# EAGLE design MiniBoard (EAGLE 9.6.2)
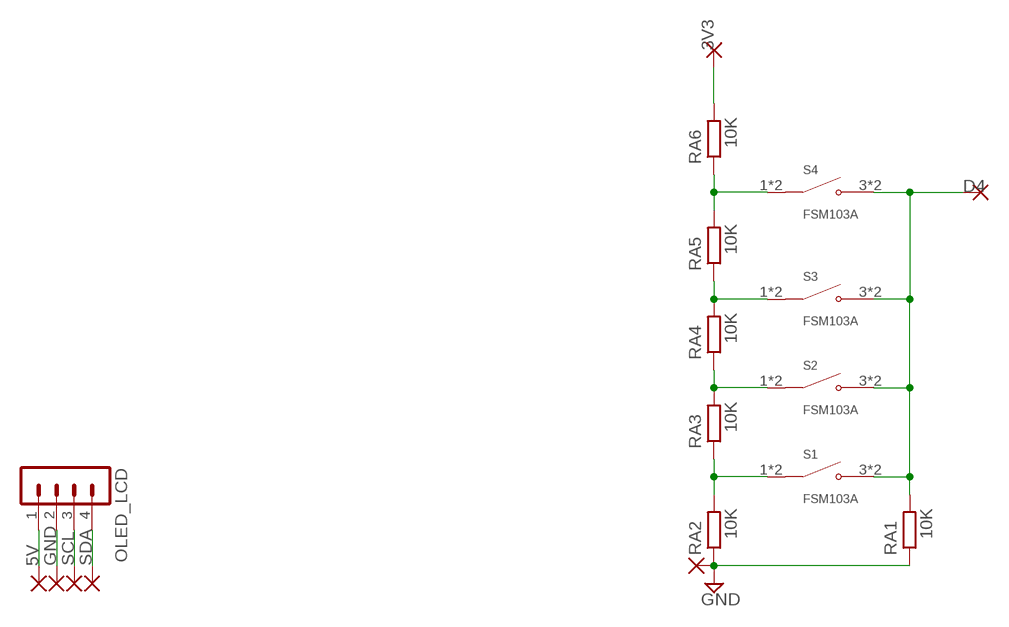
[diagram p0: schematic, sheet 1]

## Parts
OLED_LCD  MA04-1  [MA04-1]
PAD1  WIREPAD1,6/0,9  [1,6/0,9]
PAD25  WIREPAD1,6/0,9  [1,6/0,9]
PAD26  WIREPAD1,6/0,9  [1,6/0,9]
PAD52  WIREPAD1,6/0,9  [1,6/0,9]
PAD78  WIREPAD1,6/0,9  [1,6/0,9]
PAD103  WIREPAD1,6/0,9  [1,6/0,9]
PAD104  WIREPAD1,6/0,9  [1,6/0,9]
RA1  10K  R-EU_0309/12  [0309/12]
RA2  10K  R-EU_0309/12  [0309/12]
RA3  10K  R-EU_0309/12  [0309/12]
RA4  10K  R-EU_0309/12  [0309/12]
RA5  10K  R-EU_0309/12  [0309/12]
RA6  10K  R-EU_0309/12  [0309/12]
S1  FSM103A  [SW_1571627-1]
S2  FSM103A  [SW_1571627-1]
S3  FSM103A  [SW_1571627-1]
S4  FSM103A  [SW_1571627-1]

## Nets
3V3: PAD104.1(P) RA6.2
5V: OLED_LCD.1 PAD25.1(P)
D4: PAD103.1(P) RA1.2 S1.3(NO) S1.4(NO) S2.3(NO) S2.4(NO) S3.3(NO) S3.4(NO) S4.3(NO) S4.4(NO)
GND: OLED_LCD.2 PAD1.1(P) PAD26.1(P) RA1.1 RA2.1
N$5: RA4.2 RA5.1 S3.1(COM) S3.2(COM)
N$8: RA3.2 RA4.1 S2.1(COM) S2.2(COM)
N$9: RA2.2 RA3.1 S1.1(COM) S1.2(COM)
N$32: RA5.2 RA6.1 S4.1(COM) S4.2(COM)
SCL: OLED_LCD.3 PAD52.1(P)
SDA: OLED_LCD.4 PAD78.1(P)

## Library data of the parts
OLED_LCD = con-lstb:MA04-1: PIN HEADER; OC_FARNELL: unknown; OC_NEWARK: unknown
PAD1 PAD25 PAD26 PAD52 PAD78 PAD103 PAD104 = wirepad-ws:WIREPAD: Wire PAD connect wire on PCB
RA1-RA6 = rcl-ws:R-EU_: RESISTOR, European symbol; SPICEPREFIX: R
S1-S4 = FSM103A:FSM103A: Alcoswitch FSM100-104, Tactile Switches, Round Actuator Style, Operating Function NO, Brass Contact Base Material Check availability; AVAILABILITY: In Stock; CHECK_PRICES: https://www.snapeda.com/parts/FSM103A/TE+Connectivity+ALCOSWITCH+Switches/view-part/?ref=eda; COMMENT: 1571627-1; DESCRIPTION: Alcoswitch, Tactile switch,PCB,SPST,red actuator | TE Connectivity FSM103A; MF: TE Connectivity; MP: FSM103A; PACKAGE: None; PRICE: None; SNAPEDA_LINK: https://www.snapeda.com/parts/FSM103A/TE+Connectivity+ALCOSWITCH+Switches/view-part/?ref=snap

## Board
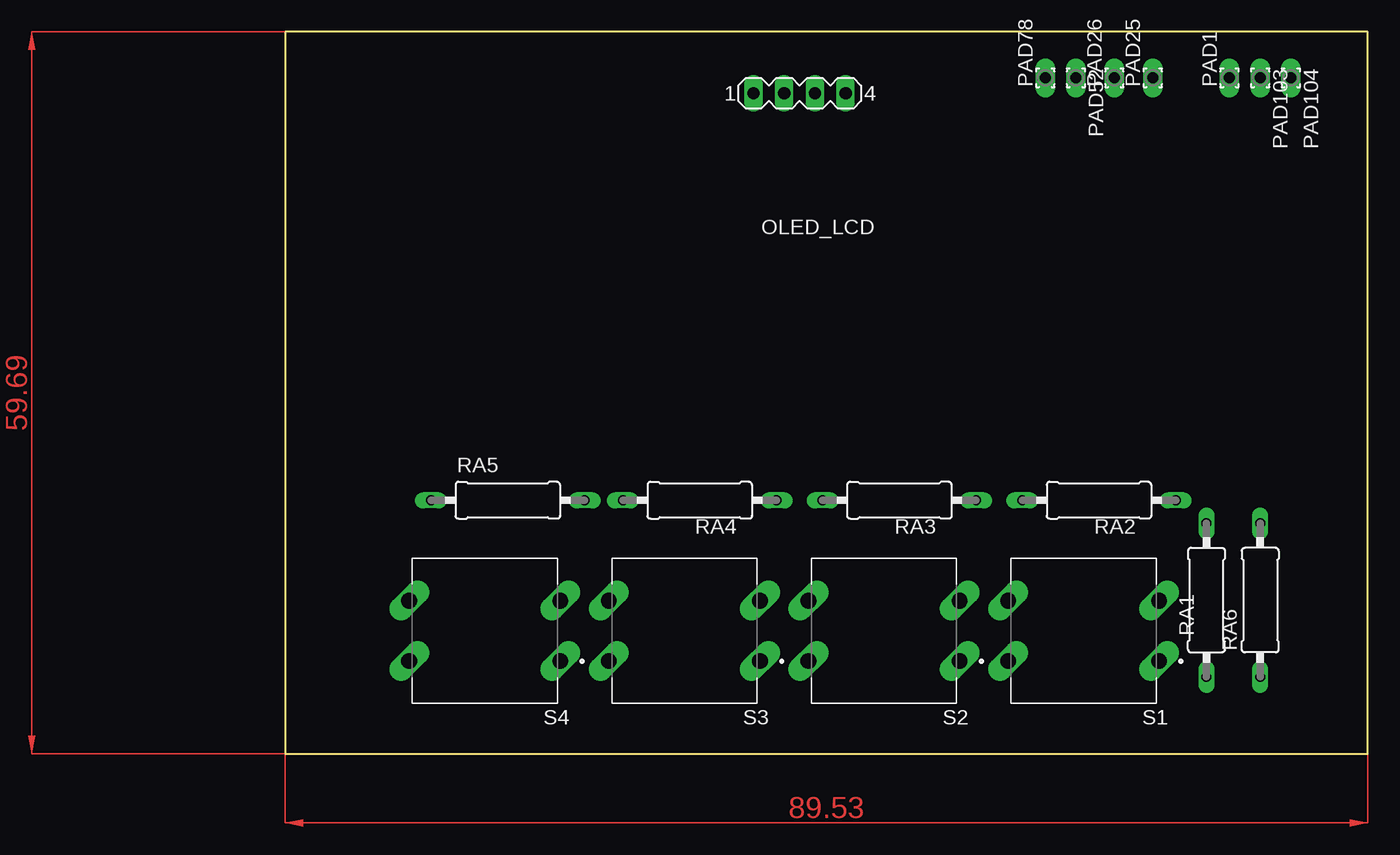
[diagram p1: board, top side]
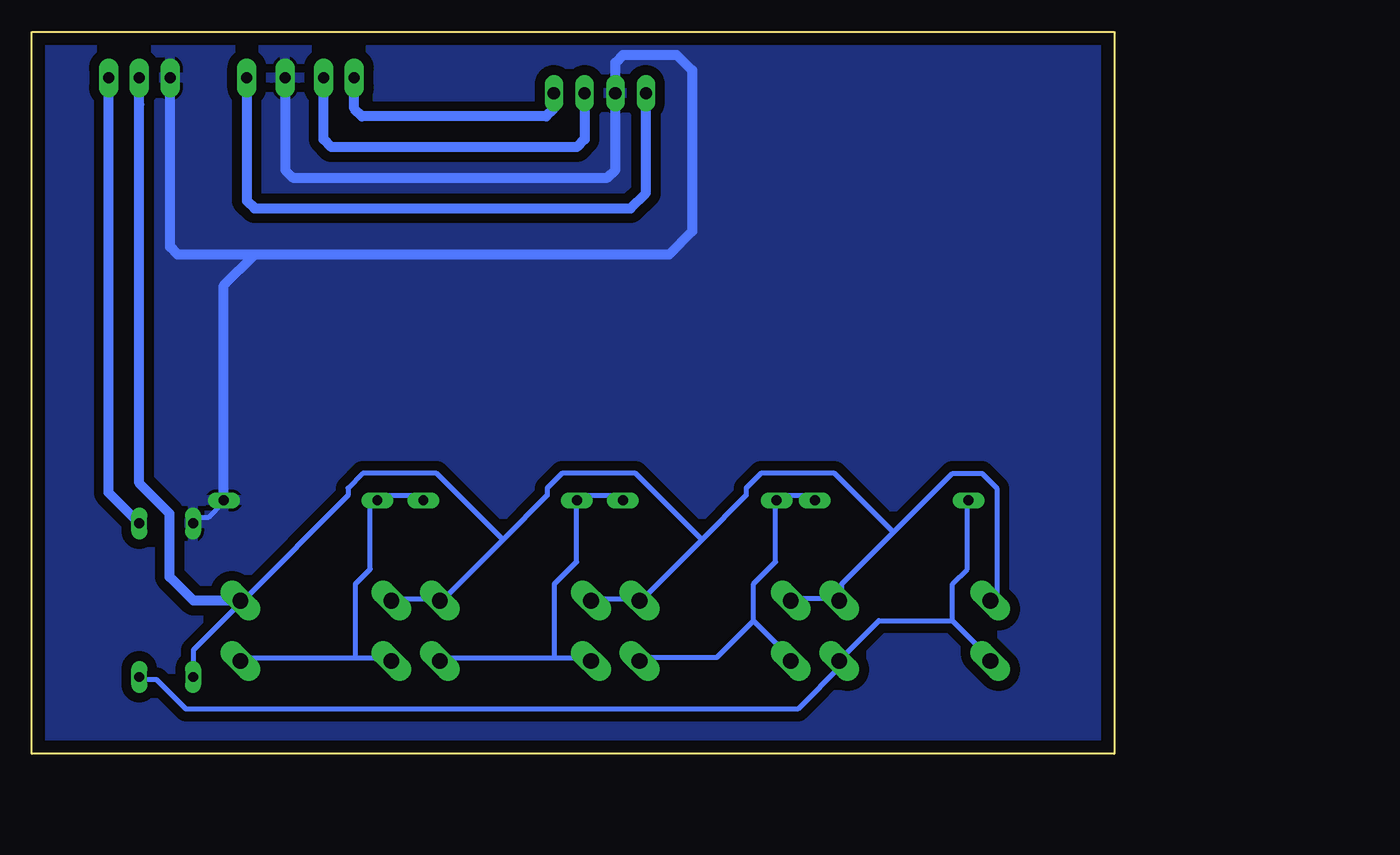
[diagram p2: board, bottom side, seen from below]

Size 89.53 x 59.69 mm. Coordinates in mm from the lower left corner, seen from the top.
Outline: 0,0 89.53,0 89.53,59.69 0,59.69 0,0
Copper layers (1*16): Top 0.035mm / dielectric 1.5mm / Bottom 0.035mm
Design rules "default *": minimum track width 16mil, minimum drill 0.35mm, track to track 32mil, track to pad 32mil, pad to pad 32mil, via to via 32mil, smd to smd 6mil, copper to edge 40mil, drill to drill 6mil, minimum pad ring 10mil, minimum via ring 8mil, stop-mask expansion 4mil, vias tented up to drill 0mil, thermal gap 10mil

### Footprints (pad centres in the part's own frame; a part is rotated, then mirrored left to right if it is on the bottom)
MA04-1 = drill 1.016 long: 1 -3.81,0; 2 -1.27,0; 3 1.27,0; 4 3.81,0
1,6/0,9 = drill 0.914 pad 1.6 long: 1 0,0
0309/12 = drill 0.813 long: 1 -6.35,0; 2 6.35,0
SW_1571627-1 = drill 1.3 long: 1 -6.25,2.5; 2 6.25,2.5; 3 -6.25,-2.5; 4 6.25,-2.5

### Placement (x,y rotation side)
OLED_LCD  42.55,54.61 0 top
PAD1  78.1,55.88 90 top
PAD25  71.75,55.88 90 top
PAD26  68.58,55.88 90 top
PAD52  65.41,55.88 270 top
PAD78  62.87,55.88 90 top
PAD103  80.64,55.88 270 top
PAD104  83.18,55.88 270 top
RA1  76.2,12.7 270 top
RA2  67.31,20.96 180 top
RA3  50.8,20.96 180 top
RA4  34.29,20.96 180 top
RA5  18.41,20.96 180 top
RA6  80.64,12.7 90 top
S1  66.04,10.16 180 top
S2  49.53,10.16 180 top
S3  33.02,10.16 180 top
S4  16.51,10.16 180 top

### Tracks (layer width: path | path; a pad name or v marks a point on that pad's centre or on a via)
3V3
  Bottom 0.813: RA6.2 83.18,21.59 PAD104.1
5V
  Bottom 0.813: PAD25.1 71.75,45.72 71.12,45.09 40.01,45.09 38.73,46.35 OLED_LCD.1
D4
  Bottom 0.406: RA1.2 76.17,6.73 76.17,8.56 72.52,12.22 S1.3 71.91,12.83 63.37,21.36 63.37,21.97 62.15,23.19 56.06,23.19 50.57,17.7 | 80.44,53.67 80.44,55.5 PAD103.1 | S1.4 59.72,12.83 56.06,12.83 S2.3 55.45,12.83 50.57,17.7 | S2.4 43.26,12.83 39.6,12.83 S3.3 38.99,12.83 34.11,17.7 | 18.26,18.31 22.53,14.05 22.53,12.83 S4.3 23.14,12.83 26.19,12.83 S3.4 | 18.26,18.31 13.39,23.19 10.95,23.19 9.73,21.97 9.73,12.83 S4.4 | 34.11,17.7 30.45,21.36 30.45,21.97 29.23,23.19 23.14,23.19 18.26,18.31 | 50.57,17.7 46.91,21.36 46.91,21.97 45.7,23.19 39.6,23.19 34.11,17.7
  Bottom 0.813: S1.3 76.16,12.66 78.13,14.63 78.13,19.85 80.64,22.37 PAD103.1
GND
  Bottom 0.406: RA1.1 76.17,19.53 74.95,19.53 73.74,20.75 RA2.1 73.13,21.36 | 41.43,54.46 OLED_LCD.2
  Bottom 0.813: PAD26.1 68.58,48.26 67.94,47.62 41.91,47.62 41.27,48.26 OLED_LCD.2 41.27,57.15 40.64,57.78 36.2,57.78 34.93,56.52 34.93,43.18 36.83,41.27 71.12,41.27 | 71.12,41.27 77.47,41.27 78.1,41.91 PAD1.1 | RA2.1 73.66,38.73 71.12,41.27
  pour Bottom: 0,59.69 0,0 89.53,0 89.53,59.69
N$5
  Bottom 0.406: RA5.1 24.97,21.36 27.41,21.36 RA4.2 28.02,20.75 28.02,15.88 29.84,14.05 29.84,11 | 29.84,11 26.8,7.95 S3.2 | 29.84,11 32.89,7.95 38.99,7.95 S3.1
N$8
  Bottom 0.406: RA4.1 40.82,21.36 43.87,21.36 RA3.2 44.48,20.75 44.48,15.88 46.3,14.05 46.3,7.95 | 46.3,7.95 55.45,7.95 S2.1 | 46.3,7.95 43.87,7.95 S2.2
N$9
  Bottom 0.406: RA3.1 57.28,21.36 60.94,21.36 RA2.2 61.54,20.75 61.54,15.27 62.76,14.05 62.76,7.95 | 62.76,7.95 71.91,7.95 S1.1 | 62.76,7.95 60.33,7.95 S1.2
N$32
  Bottom 0.406: 13.39,11 13.39,14.05 12.17,15.27 12.17,20.75 RA5.2 | 13.39,11 10.34,7.95 S4.2 | RA6.1 80.44,6.12 79.22,6.12 76.78,3.68 26.19,3.68 22.53,7.34 S4.1 22.53,7.95 19.48,11 13.39,11
SCL
  Bottom 0.813: OLED_LCD.3 43.82,50.8 44.45,50.16 64.77,50.16 65.41,50.8 PAD52.1
SDA
  Bottom 0.813: OLED_LCD.4 46.36,53.34 46.99,52.7 62.23,52.7 62.87,53.34 PAD78.1
(copper drawn outside any net)
  shapes: Top area x2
